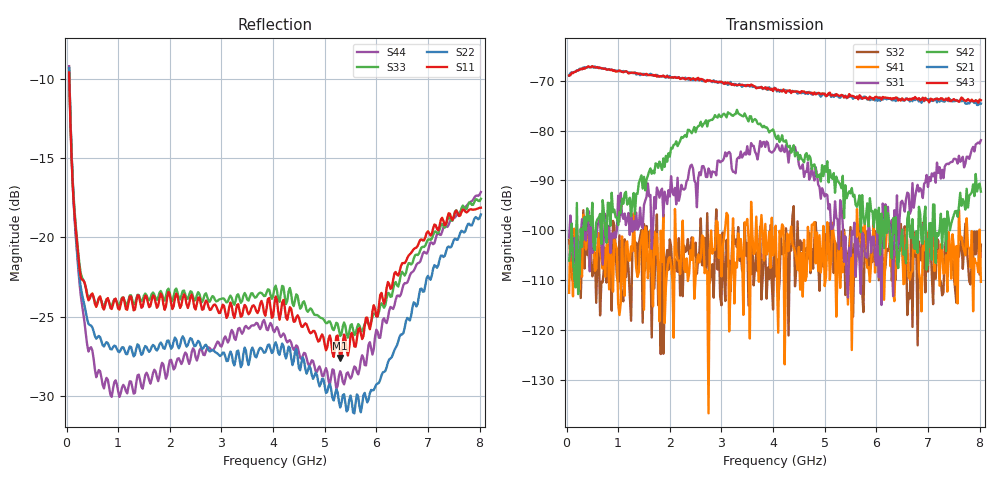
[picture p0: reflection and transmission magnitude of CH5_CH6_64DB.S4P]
!Agilent Technologies,E5071C,MY46316741,A.11.02
!Date: Mon Jun 01 10:42:28 2026
!Data & Calibration Information:
!1:CH5 INPUT 2:CH5 OUTPUT 3:CH6 INPUT 4:CH6 OUTPUT
!Freq	S11:SOLT4(ON)	S12:SOLT4(ON)	S13:SOLT4(ON)	S14:SOLT4(ON)
!	S21:SOLT4(ON)	S22:SOLT4(ON)	S23:SOLT4(ON)	S24:SOLT4(ON)
!	S31:SOLT4(ON)	S32:SOLT4(ON)	S33:SOLT4(ON)	S34:SOLT4(ON)
!	S41:SOLT4(ON)	S42:SOLT4(ON)	S43:SOLT4(ON)	S44:SOLT4(ON)
!PortZ  Port1:50+j0  Port2:50+j0  Port3:50+j0  Port4:50+j0
!Above PortZ is port z conversion or system Z0 setting when saving the data.
!When reading, reference impedance value at option line is always used.
# Hz S dB R 50
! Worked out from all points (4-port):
!   320 points, 50 MHz to 8.025 GHz, reference 50 ohm
!   strongest paths, dB at 50 MHz, 2.05 GHz, 4.05 GHz, 6.05 GHz, 8.025 GHz:
!     S43: -68.9, -69.3, -71.5, -73.4, -73.9
!     S21: -68.9, -69.3, -71.6, -73.3, -74.6
!     S42: -106.1, -83.6, -81.3, -95.5, -92.2
!     S31: -101.5, -92.3, -83.4, -109.5, -81.9
!     S41: -112.6, -110.0, -99.1, -100.3, -110.4
!     S32: -101.9, -108.5, -109.3, -110.0, -102.9
!   lowest |S11| = -27.6 dB at 5.3 GHz (marker M1), VSWR 1.09, Z = 49.5 - j4.12 ohm
!   |S11| at or under -10 dB: 53.06 MHz to end of sweep
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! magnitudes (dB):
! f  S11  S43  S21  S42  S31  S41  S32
! 50 MHz  -9.6  -68.9  -68.9  -106.1  -101.5  -112.6  -101.9
! 125 MHz  -17.0  -68.4  -68.3  -106.1  -106.2  -113.3  -109.9
! 275 MHz  -22.5  -67.6  -67.7  -99.6  -100.7  -106.8  -113.6
! 725 MHz  -24.5  -67.5  -67.5  -96.6  -100.8  -103.4  -107.7
! 3.3 GHz  -24.3  -70.8  -71.0  -75.8  -85.7  -107.5  -103.4
! 5.3 GHz  -27.6  -73.0  -73.4  -90.8  -93.9  -111.6  -109.7
! 8.025 GHz  -18.1  -73.9  -74.6  -92.2  -81.9  -110.4  -102.9
